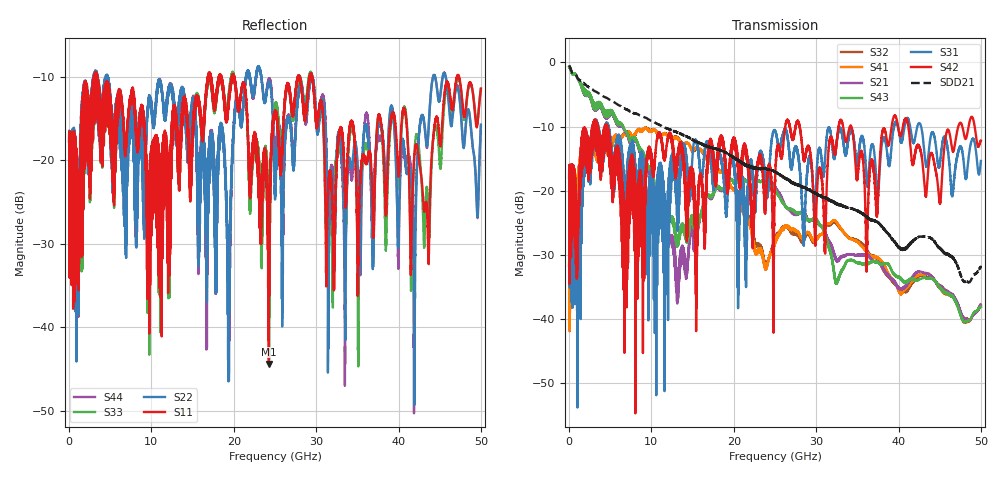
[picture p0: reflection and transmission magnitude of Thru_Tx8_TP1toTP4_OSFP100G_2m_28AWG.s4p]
! Touchstone data
! Created: 27-Feb-2019 by IdEM 12 (12.1.0)
! COMMENTS
!  Created Wed Feb 27 12:03:36 2019
!  64 Port Network Data from SP1.SP block
!  freq  magS1_1  angS1_1  magS1_2  angS1_2  magS1_3  angS1_3  magS1_4  angS1_4
!  magS1_5  angS1_5  magS1_6  angS1_6  magS1_7  angS1_7  magS1_8  angS1_8
!  magS1_9  angS1_9  magS1_10  angS1_10  magS1_11  angS1_11  magS1_12  angS1_12
!  magS1_13  angS1_13  magS1_14  angS1_14  magS1_15  angS1_15  magS1_16  angS1_16
!  magS1_17  angS1_17  magS1_18  angS1_18  magS1_19  angS1_19  magS1_20  angS1_20
!  magS1_21  angS1_21  magS1_22  angS1_22  magS1_23  angS1_23  magS1_24  angS1_24
!  magS1_25  angS1_25  magS1_26  angS1_26  magS1_27  angS1_27  magS1_28  angS1_28
!  magS1_29  angS1_29  magS1_30  angS1_30  magS1_31  angS1_31  magS1_32  angS1_32
!  magS1_33  angS1_33  magS1_34  angS1_34  magS1_35  angS1_35  magS1_36  angS1_36
!  magS1_37  angS1_37  magS1_38  angS1_38  magS1_39  angS1_39  magS1_40  angS1_40
!  magS1_41  angS1_41  magS1_42  angS1_42  magS1_43  angS1_43  magS1_44  angS1_44
!  magS1_45  angS1_45  magS1_46  angS1_46  magS1_47  angS1_47  magS1_48  angS1_48
!  magS1_49  angS1_49  magS1_50  angS1_50  magS1_51  angS1_51  magS1_52  angS1_52
!  magS1_53  angS1_53  magS1_54  angS1_54  magS1_55  angS1_55  magS1_56  angS1_56
!  magS1_57  angS1_57  magS1_58  angS1_58  magS1_59  angS1_59  magS1_60  angS1_60
!  magS1_61  angS1_61  magS1_62  angS1_62  magS1_63  angS1_63  magS1_64  angS1_64
!  magS2_1  angS2_1  magS2_2  angS2_2  magS2_3  angS2_3  magS2_4  angS2_4
!  magS2_5  angS2_5  magS2_6  angS2_6  magS2_7  angS2_7  magS2_8  angS2_8
!  magS2_9  angS2_9  magS2_10  angS2_10  magS2_11  angS2_11  magS2_12  angS2_12
!  magS2_13  angS2_13  magS2_14  angS2_14  magS2_15  angS2_15  magS2_16  angS2_16
!  magS2_17  angS2_17  magS2_18  angS2_18  magS2_19  angS2_19  magS2_20  angS2_20
!  magS2_21  angS2_21  magS2_22  angS2_22  magS2_23  angS2_23  magS2_24  angS2_24
!  magS2_25  angS2_25  magS2_26  angS2_26  magS2_27  angS2_27  magS2_28  angS2_28
!  magS2_29  angS2_29  magS2_30  angS2_30  magS2_31  angS2_31  magS2_32  angS2_32
!  magS2_33  angS2_33  magS2_34  angS2_34  magS2_35  angS2_35  magS2_36  angS2_36
!  magS2_37  angS2_37  magS2_38  angS2_38  magS2_39  angS2_39  magS2_40  angS2_40
!  magS2_41  angS2_41  magS2_42  angS2_42  magS2_43  angS2_43  magS2_44  angS2_44
!  magS2_45  angS2_45  magS2_46  angS2_46  magS2_47  angS2_47  magS2_48  angS2_48
!  magS2_49  angS2_49  magS2_50  angS2_50  magS2_51  angS2_51  magS2_52  angS2_52
!  magS2_53  angS2_53  magS2_54  angS2_54  magS2_55  angS2_55  magS2_56  angS2_56
!  magS2_57  angS2_57  magS2_58  angS2_58  magS2_59  angS2_59  magS2_60  angS2_60
!  magS2_61  angS2_61  magS2_62  angS2_62  magS2_63  angS2_63  magS2_64  angS2_64
!  magS3_1  angS3_1  magS3_2  angS3_2  magS3_3  angS3_3  magS3_4  angS3_4
!  magS3_5  angS3_5  magS3_6  angS3_6  magS3_7  angS3_7  magS3_8  angS3_8
!  magS3_9  angS3_9  magS3_10  angS3_10  magS3_11  angS3_11  magS3_12  angS3_12
!  magS3_13  angS3_13  magS3_14  angS3_14  magS3_15  angS3_15  magS3_16  angS3_16
!  magS3_17  angS3_17  magS3_18  angS3_18  magS3_19  angS3_19  magS3_20  angS3_20
!  magS3_21  angS3_21  magS3_22  angS3_22  magS3_23  angS3_23  magS3_24  angS3_24
!  magS3_25  angS3_25  magS3_26  angS3_26  magS3_27  angS3_27  magS3_28  angS3_28
!  magS3_29  angS3_29  magS3_30  angS3_30  magS3_31  angS3_31  magS3_32  angS3_32
!  magS3_33  angS3_33  magS3_34  angS3_34  magS3_35  angS3_35  magS3_36  angS3_36
!  magS3_37  angS3_37  magS3_38  angS3_38  magS3_39  angS3_39  magS3_40  angS3_40
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# Hz S MA R 50
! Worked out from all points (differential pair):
!   5000 points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, 10 MHz to 50 GHz, reference 50 ohm
!   strongest paths, dB at 10 MHz, 12.51 GHz, 25.01 GHz, 37.51 GHz, 50 GHz:
!     S42: -18.0, -12.2, -18.3, -20.7, -12.2
!     S31: -18.0, -15.9, -10.7, -20.7, -15.4
!     S43: -0.7, -24.4, -19.8, -31.3, -38.1
!     S21: -0.7, -27.8, -19.3, -31.2, -37.8
!     S41: -31.7, -12.0, -28.3, -30.6, -37.8
!     S32: -31.7, -11.9, -27.7, -31.0, -38.1
!   taken as a pair (ports 3,1 in; 4,2 out), SDD21 dB: -0.5, -10.6, -17.1, -25.0, -32.0
!   lowest |S11| = -44.4 dB at 24.26 GHz (marker M1), VSWR 1.01, Z = 49.6 - j0.401 ohm
!   |S11| at or under -10 dB: 3.451 GHz to 16.86 GHz (13.4 GHz wide, 132 % of centre); 20.09 GHz to 27.79 GHz (7.695 GHz wide, 32.1 % of centre); 29.5 GHz to 47.1 GHz (17.61 GHz wide, 46 % of centre)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
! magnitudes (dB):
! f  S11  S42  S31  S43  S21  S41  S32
! 10 MHz  -17.7  -18.0  -18.0  -0.7  -0.7  -31.7  -31.7
! 1.58 GHz  -14.2  -11.4  -12.1  -3.9  -4.0  -14.8  -14.8
! 13.16 GHz  -17.4  -14.6  -19.7  -27.4  -33.7  -11.9  -11.8
! 19.38 GHz  -12.7  -17.2  -18.2  -18.2  -18.1  -18.3  -18.4
! 24.26 GHz  -44.4  -16.4  -18.3  -18.8  -18.4  -30.7  -30.6
! 33.48 GHz  -23.2  -11.8  -14.1  -31.6  -30.1  -26.6  -26.7
! 50 GHz  -11.4  -12.2  -15.4  -38.1  -37.8  -37.8  -38.1
